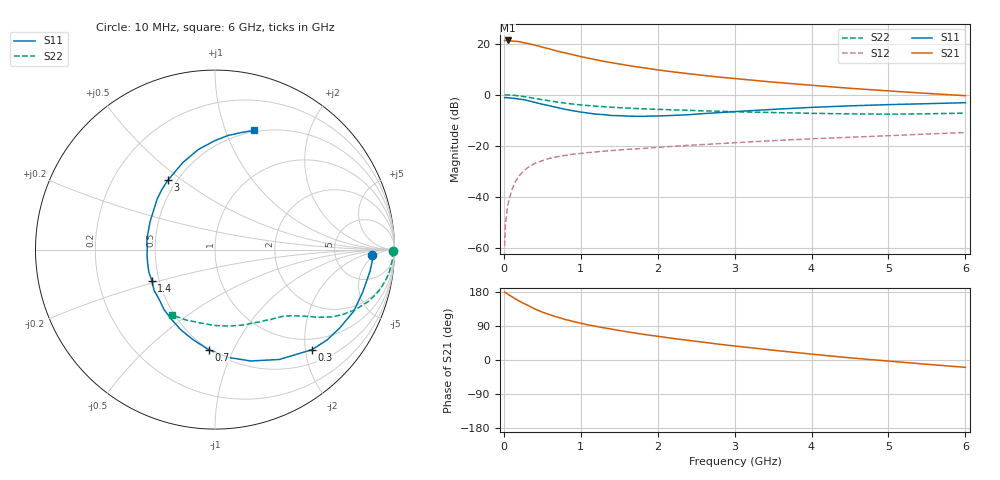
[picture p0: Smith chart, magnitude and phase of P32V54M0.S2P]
! SIEMENS Small Signal Semiconductors
! BFP181
! Si NPN RF Bipolar Junction Transistor in SOT143
! VCE = 2.5 V  IC = 4 mA
! Common Emitter S-Parameters:  March  1996
# GHz  S  MA  R  50
!  f  S11  S21  S12  S22
! GHz  MAG  ANG  MAG  ANG  MAG  ANG  MAG  ANG
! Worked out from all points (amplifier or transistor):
!   36 points, 10 MHz to 6 GHz, reference 50 ohm
!   highest |S21| = 21.2 dB at 50 MHz (marker M1)
!   |S21| within 3 dB of that: start of sweep to 552.2 MHz
!   unconditionally stable (mu >= 1): 1.796 GHz to end of sweep
!   at 250 MHz: K = 0.19, MSG = 25.2 dB, |S12| = -30.1 dB
!   at 1.4 GHz: K = 0.86, MSG = 17.2 dB, |S12| = -21.8 dB
!   at 6 GHz: K = 1.06, MAG = 5.7 dB, |S12| = -14.8 dB
!   S11 on the Smith chart (normalised r, x): 10 MHz: 14, -3; 300 MHz: 0.76, -2.13; 700 MHz: 0.50, -0.81; 1.4 GHz: 0.46, -0.19; 3 GHz: 0.45, +0.44; 6 GHz: 0.49, +1.26
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0.01  0.8746 -1.9  11.43 178.8  0.0011 78.6  0.9917 -0.6
0.02  0.8803 -3.3  11.45 177.9  0.0029 81.9  0.9905 -1.3
0.05  0.8722 -7.9  11.48 173.8  0.0068 87.3  0.989 -3.5
0.15  0.8458 -23.9  11.07 161.4  0.0201 76.5  0.9655 -10.2
0.2  0.8214 -31.9  10.86 155.6  0.0262 72.8  0.9467 -13.5
0.25  0.8022 -38.9  10.41 150.1  0.0314 69.1  0.9234 -16.3
0.3  0.7758 -46.0  10.09 145.4  0.0367 65.7  0.9004 -18.8
0.4  0.7096 -59.6  9.353 134.9  0.0453 59.0  0.8487 -23.3
0.5  0.6518 -72.2  8.506 126.4  0.0515 53.5  0.7986 -26.9
0.6  0.6055 -82.9  7.791 119.3  0.0574 50.3  0.7556 -29.7
0.7  0.5587 -93.6  7.062 112.9  0.0617 47.2  0.7171 -31.7
0.8  0.517 -103.6  6.542 106.9  0.0654 44.2  0.685 -33.4
0.9  0.4858 -113.1  6.031 101.8  0.069 42.3  0.6552 -34.8
1.1  0.4377 -130.6  5.18 92.5  0.0741 39.4  0.6122 -37.2
1.4  0.392 -153.9  4.222 81.5  0.081 36.8  0.5699 -40.4
1.8  0.3775 178.3  3.378 68.2  0.089 35.3  0.5308 -44.5
2.2  0.394 156.5  2.793 56.9  0.098 33.5  0.5056 -49.4
3  0.4676 124.1  2.071 37.0  0.1153 30.5  0.4647 -61.0
3.5  0.5174 110.2  1.763 25.9  0.1266 28.3  0.4483 -69.6
4.5  0.6058 90.3  1.335 5.7  0.1477 22.8  0.4229 -90.3
5.5  0.6679 77.4  1.061 -11.3  0.1707 17.8  0.4241 -112.4
6  0.6987 71.9  0.958 -19.4  0.1827 14.4  0.4366 -123.7
